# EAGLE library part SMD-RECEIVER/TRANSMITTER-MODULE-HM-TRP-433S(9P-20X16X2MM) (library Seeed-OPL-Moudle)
317070000
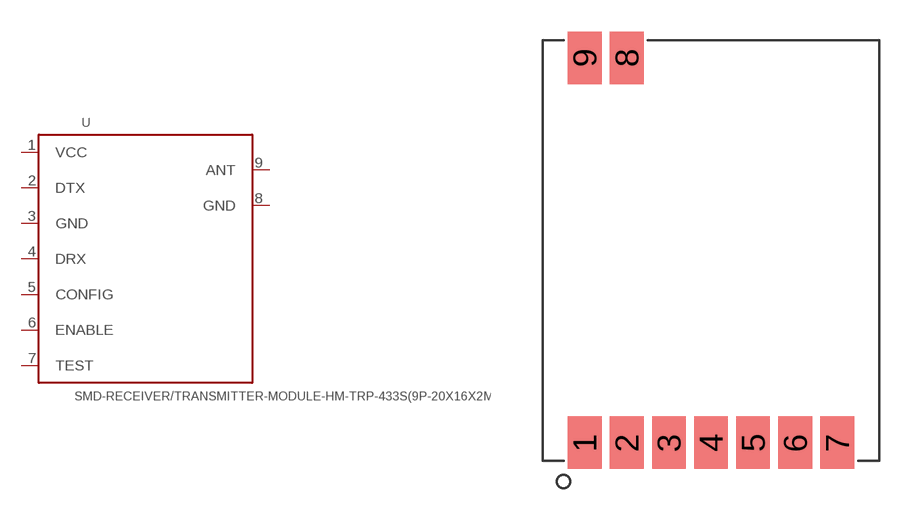
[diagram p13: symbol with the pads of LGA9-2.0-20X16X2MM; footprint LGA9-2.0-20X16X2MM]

Designator prefix U

## SMD-RECEIVER/TRANSMITTER-MODULE-HM-TRP-433S(9P-20X16X2MM) (MPN: HM-TRP-433S; VALUE: HM-TRP-433S)  [LGA9-2.0-20X16X2MM]
1  VCC  pwr
2  DTX
3  GND  sup
4  DRX
5  CONFIG
6  ENABLE
7  TEST
8  GND
9  ANT

## Footprint LGA9-2.0-20X16X2MM (pad centres in mm)
smd 1.6 x 2.5: 1 -6,-9.15; 2 -4,-9.15; 3 -2,-9.15; 4 0,-9.15; 5 2,-9.15; 6 4,-9.15; 7 6,-9.15; 8 -4,9.15; 9 -6,9.15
